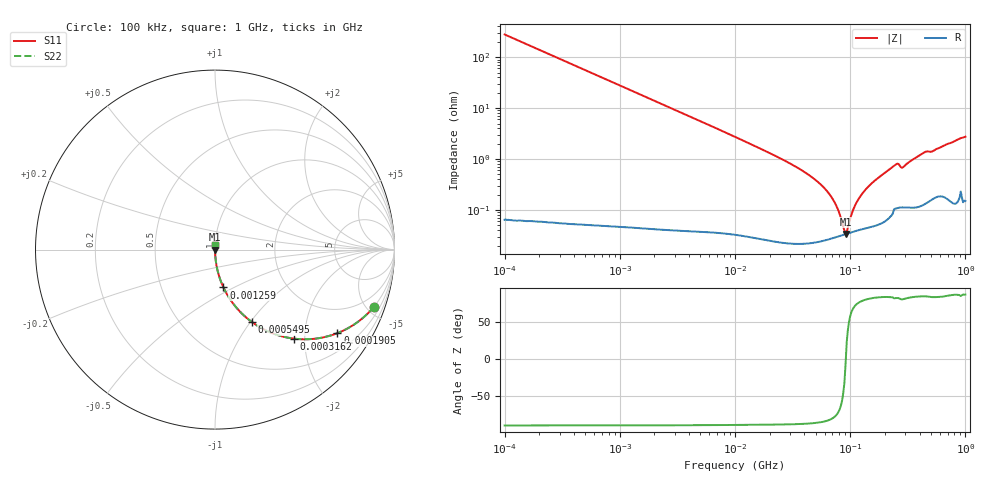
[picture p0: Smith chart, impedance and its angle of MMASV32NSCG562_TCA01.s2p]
! MMASV32NSCG562_TCA01  S-PARAMETER MODEL  ( Standard Model )
! Model Generated by TAIYO YUDEN Corporation (https://www.yuden.co.jp/en/)
! Version 1.0
! TAIYO YUDEN Control No. 250312
! Copyright(c) 2025 TAIYO YUDEN CO.,LTD. All Rights Reserved.
! Product Description (link to TY-COMPAS)
! https://ds.yuden.co.jp/TYCOMPAS/or/detail?pn=MMASV32NSCG562JTCA01&u=M
! Products Name : Multilayer Ceramic Capacitors
! Characteristics :
!  Capacitance : 5600 [pF] , Rated Voltage : 1000 [V] , TCC : CG / C0G
!  Case Size : 3.2 x 2.5 / 0.126 x 0.098 [mm/inch] , Thickness : 1.9 / 0.075 [mm/inch]
!  (Conditions: Temperature = 25 [degC] , DC Bias Voltage = 0 [V])
! External Node Assignments :
!  1  o---| |---o  2
! GND o---------o GND
! Frequency Range : 0.1MHz  -  1000MHz  [ 401 STEP ]
# MHZ S RI R 50
! Freq[MHz].  S11 Real  S11 Imag  S21 Real  S21 Imag  S12 Real  S12 Imag  S22 Real  S22 Imag
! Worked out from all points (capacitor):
!   401 points, 100 kHz to 1 GHz, reference 50 ohm
!   read as one part in series: C = 5.71 nF near 104.7 kHz
!   lowest |Z| = 34.1 mohm at 91.2 MHz (marker M1)
!   series resonance near 91.64 MHz, so ESL is about 530 pH
!   S11 on the Smith chart (normalised r, x): 100 kHz: 1.00, -5.58; 190.5 kHz: 1.00, -2.93; 316.2 kHz: 1.00, -1.77; 549.5 kHz: 1.00, -1.02; 1.259 MHz: 1.00, -0.44; 1 GHz: 1.00, +0.06
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0.1  0.8861 -0.3176  0.1139 0.3176  0.1139 0.3176  0.8861 -0.3176
0.190546  0.6822 -0.4654  0.3178 0.4654  0.3178 0.4654  0.6822 -0.4654
0.316228  0.4379 -0.4958  0.5621 0.4958  0.5621 0.4958  0.4379 -0.4958
0.467735  0.2628 -0.4397  0.7372 0.4397  0.7372 0.4397  0.2628 -0.4397
0.549541  0.2054 -0.4035  0.7946 0.4035  0.7946 0.4035  0.2054 -0.4035
1.258925  0.0472 -0.2111  0.9528 0.2111  0.9528 0.2111  0.0472 -0.2111
2.187762  0.0164 -0.1254  0.9836 0.1254  0.9836 0.1254  0.0164 -0.1254
10  0.00108 -0.0273  0.9989 0.0273  0.9989 0.0273  0.00108 -0.0273
26.91535  0.000314 -0.00938  0.9997 0.00938  0.9997 0.00938  0.000314 -0.00938
46.77351  0.000246 -0.00438  0.9998 0.00438  0.9998 0.00438  0.000246 -0.00438
69.1831  0.000281 -0.00174  0.9997 0.00174  0.9997 0.00174  0.000281 -0.00174
77.62471  0.000302 -0.00103  0.9997 0.00103  0.9997 0.00103  0.000302 -0.00103
87.09636  0.000328 -0.000338  0.9997 0.000338  0.9997 0.000338  0.000328 -0.000338
91.20108  0.000339 -3.76e-05  0.9997 3.76e-05  0.9997 3.76e-05  0.000339 -3.76e-05
95.49926  0.000351 0.000288  0.9996 -0.000288  0.9996 -0.000288  0.000351 0.000288
109.6478  0.000387 0.00114  0.9996 -0.00114  0.9996 -0.00114  0.000387 0.00114
125.8925  0.000423 0.00199  0.9996 -0.00199  0.9996 -0.00199  0.000423 0.00199
218.7762  0.000745 0.00621  0.9993 -0.00621  0.9993 -0.00621  0.000745 0.00621
251.1886  0.00114 0.00788  0.9989 -0.00788  0.9989 -0.00788  0.00114 0.00788
288.4031  0.00118 0.00686  0.9988 -0.00686  0.9988 -0.00686  0.00118 0.00686
436.5158  0.00145 0.0133  0.9985 -0.0133  0.9985 -0.0133  0.00145 0.0133
1000  0.00226 0.0274  0.9977 -0.0274  0.9977 -0.0274  0.00226 0.0274
